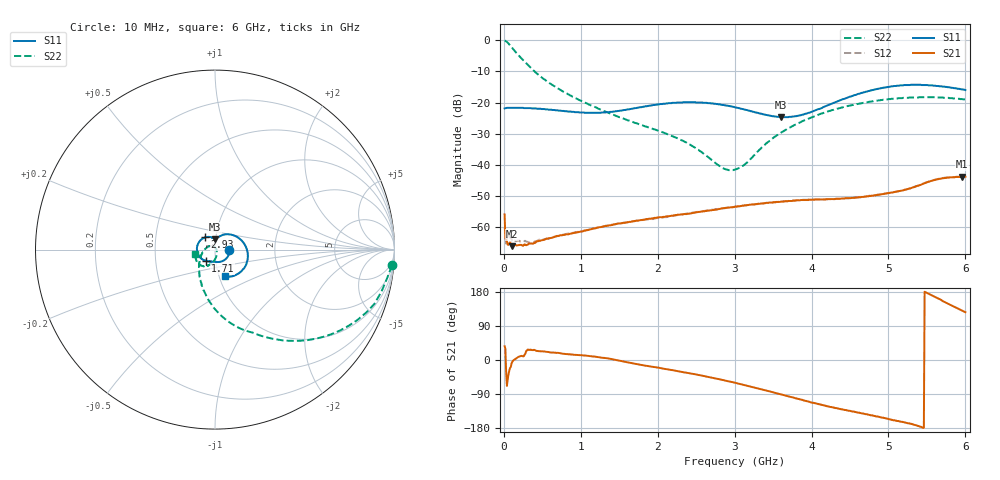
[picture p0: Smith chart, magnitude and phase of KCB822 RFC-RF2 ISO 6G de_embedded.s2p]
!Agilent	"Technologies,N5230A,MY45001650,A.07.50.48"
!Agilent	N5230A:	A.07.50.48
!Date:	"Wednesday,"	February	"12,"	2014	15:16:38
!Correction:	S11(Full	2	"Port(1,2))"
!S21(Full	2	"Port(1,2))"
!S12(Full	2	"Port(1,2))"
!S22(Full	2	"Port(1,2))"
!S2P	File:	Measurements:	"S11,"	"S21,"	"S12,"	S22:
#	Hz	S	dB	R	50
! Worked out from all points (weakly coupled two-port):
!   600 points, 10 MHz to 6 GHz, reference 50 ohm
!   highest |S21| = -43.80 dB at 5.96 GHz (marker M1); lowest = -66.1 dB at 100 MHz (marker M2)
!   lowest |S11| = -24.7 dB at 3.6 GHz (marker M3), VSWR 1.12, Z = 49.8 + j5.82 ohm
!   |S11| at or under -10 dB: start of sweep to end of sweep
!   |S22| runs from -41.7 to -0.1 dB; largest |S21 - S12| = 0.0014
!   S11 on the Smith chart (normalised r, x): 10 MHz: 1.17, -0.01; 1.71 GHz: 0.89, -0.11; 2.93 GHz: 0.89, +0.12; 6 GHz: 1.06, -0.32
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1e7  -21.90 -1.7  -55.90 36.3  -59.90 -20.8  -0.09 -5.1
5e7  -21.70 -4.8  -65.60 -52.2  -62.80 12.5  -0.79 -22.6
1e8  -21.70 -8.8  -66.10 -9.2  -63.80 34.8  -2.23 -39.0
2.1e8  -21.70 -18.9  -65.70 9.6  -64.60 28.6  -5.36 -62.4
3.7e8  -21.90 -33.7  -65.30 26.3  -64.80 25.3  -9.37 -88.9
6.3e8  -22.40 -57.4  -63.40 19.9  -63.30 20.1  -14.40 -115.0
1.01e9  -23.20 -86.6  -61.40 12.6  -61.30 12.9  -19.50 -144.0
1.71e9  -21.80 -130.0  -58.00 -9.9  -58.00 -8.6  -26.60 166.0
2.01e9  -20.60 -152.0  -56.90 -20.2  -57.00 -19.0  -29.10 146.0
2.39e9  -19.90 176.0  -55.70 -34.1  -55.60 -33.3  -33.10 122.0
2.81e9  -20.60 140.0  -54.10 -51.1  -54.10 -50.6  -40.50 67.3
2.93e9  -21.10 129.0  -53.70 -56.7  -53.70 -56.4  -41.70 35.2
3.01e9  -21.60 123.0  -53.40 -60.3  -53.40 -60.1  -41.50 12.3
3.13e9  -22.30 114.0  -53.00 -66.1  -53.00 -66.1  -39.90 -19.6
3.6e9  -24.70 88.6  -51.80 -90.7  -51.80 -90.3  -29.70 -74.2
4.01e9  -22.90 75.0  -51.20 -113.0  -51.10 -113.0  -24.70 -92.4
4.53e9  -17.90 39.5  -50.60 -136.0  -50.60 -136.0  -20.80 -110.0
5.01e9  -15.00 -1.0  -49.00 -156.0  -49.00 -156.0  -18.90 -126.0
5.39e9  -14.30 -31.4  -46.70 -174.0  -46.60 -174.0  -18.40 -139.0
5.68e9  -14.80 -51.8  -44.40 159.0  -44.30 158.0  -18.40 -151.0
5.96e9  -15.80 -68.2  -43.80 130.0  -43.80 130.0  -18.90 -165.0
6e9  -16.00 -70.2  -43.80 126.0  -43.70 126.0  -19.00 -167.0
